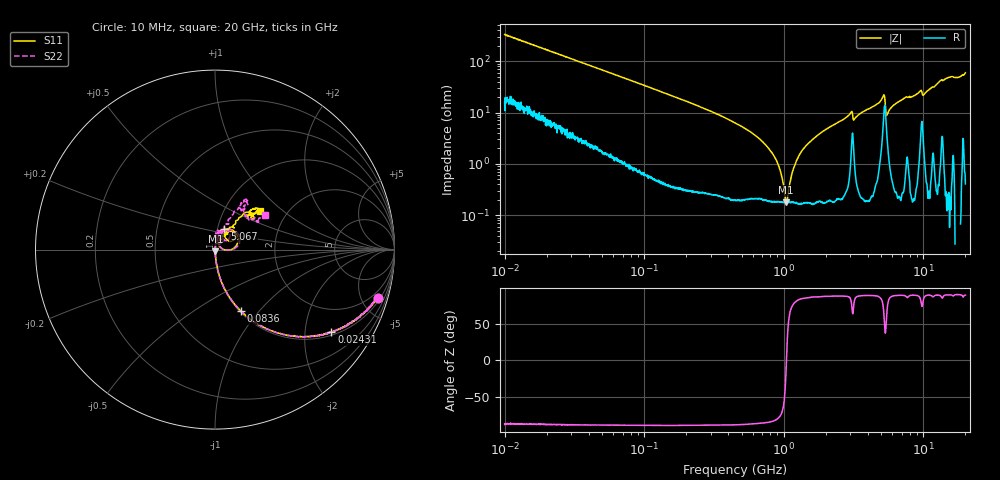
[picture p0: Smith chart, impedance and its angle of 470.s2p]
!Keysight Technologies,P5008B,MY61100088,A.16.20.02
!Date: Friday, August 30, 2024 14:14:49
!Correction: S11(C  2-Port  )
!S21(C  2-Port  )
!S12(C  2-Port  )
!S22(C  2-Port  )
!S2P File: Measurements: S11, S21, S12, S22:Log Frequency Sweep
# Hz S  MA  R 50
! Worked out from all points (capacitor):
!   1601 points, 10 MHz to 20 GHz, reference 50 ohm
!   read as one part in series: C = 48.1 pF near 10.39 MHz
!   lowest |Z| = 179 mohm at 1.042 GHz (marker M1)
!   series resonance near 1.044 GHz, so ESL is about 480 pH
!   S11 on the Smith chart (normalised r, x): 10 MHz: 1.30, -6.62; 24.31 MHz: 1.11, -2.75; 83.6 MHz: 1.01, -0.81; 5.067 GHz: 1.08, +0.25; 20 GHz: 1.47, +0.72
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1e7  0.9457 -16.6  0.2853 70.7  0.2853 70.7  0.9451 -16.6
2.431128e7  0.7937 -35.2  0.5772 52.4  0.5773 52.4  0.7933 -35.3
3.555162e7  0.677 -45.7  0.7156 42.6  0.7156 42.6  0.677 -45.7
8.360365e7  0.3735 -67.0  0.9205 21.8  0.9204 21.8  0.3735 -67.1
1.263918e8  0.2583 -74.2  0.9616 14.8  0.9614 14.8  0.2583 -74.3
4.472136e8  0.06721 -84.5  0.9957 3.4  0.9954 3.4  0.06713 -85.7
8.137127e8  0.02475 -83.5  0.9977 0.5  0.9976 0.5  0.02463 -87.9
1.041729e9  0.009803 -73.7  0.9981 -0.5  0.9979 -0.5  0.00939 -88.1
1.129349e9  0.005984 -51.7  0.9982 -0.9  0.998 -0.9  0.004689 -96.1
1.189933e9  0.004122 -21.7  0.9982 -1.1  0.9981 -1.1  0.001774 -112.6
1.224338e9  0.003664 3.5  0.9982 -1.2  0.998 -1.2  0.0004625 158.6
1.352781e9  0.006917 72.6  0.9982 -1.7  0.998 -1.7  0.006787 79.2
1.589917e9  0.01515 78.0  0.9983 -2.5  0.998 -2.5  0.01466 85.4
2.990698e9  0.06386 76.8  0.9904 -7.2  0.9903 -7.2  0.0635 74.5
3.257685e9  0.04487 80.1  0.9933 -6.4  0.9929 -6.4  0.04526 71.5
5.067356e9  0.1243 65.3  0.9656 -13.9  0.9654 -14.0  0.1266 61.1
5.213871e9  0.1488 41.7  0.9046 -14.2  0.9044 -14.3  0.1551 37.4
5.652411e9  0.03761 58.8  0.988 -10.1  0.9878 -10.2  0.04007 59.6
7.375132e9  0.1033 56.9  0.9931 -16.4  0.9932 -16.5  0.1017 82.5
1.018741e10  0.09032 52.1  0.9884 -21.7  0.9881 -21.8  0.08401 65.6
1.341918e10  0.2804 48.0  0.9514 -32.6  0.9512 -32.7  0.2735 57.1
2e10  0.3333 40.7  0.9421 -51.4  0.9419 -51.6  0.3398 34.9
